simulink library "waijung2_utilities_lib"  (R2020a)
settings: Solver=VariableStepAuto  StartTime=0.0  StopTime=10.0  RelTol=1e-3
InitFcn:
  | waijung2_host_setup
undefined symbols (not defined in the file): BasicCustomCode, Button1, CircularBuffer, DataBuffer, fcn_call, float, int32_t, IRQ, IRQCustomCode, IRQCustomCode_ISR, OutputtoState, pointer_var, PointerBlock, Print, processing, Sensor1, Sensor2, Setup, statename, StringProcessing, Switch1, Switch2, Vector3x1, void

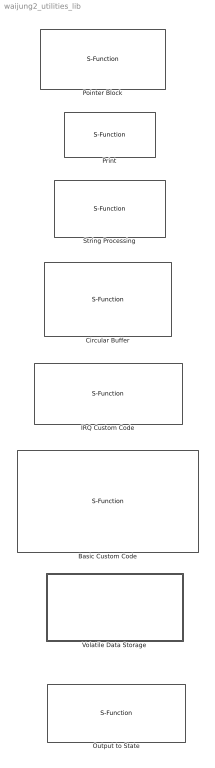
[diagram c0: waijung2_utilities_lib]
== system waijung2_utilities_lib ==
  Basic Custom Code : S-Function  FunctionName=waijung2_basic_customcode  Parameters=blockid,inputportcount,outputportcount,inputportdiminfo,outputportdiminfo,initialfuncallstr,enablefuncallstr,outputfuncallstr,disablefuncallstr,cinputportlabelstr,coutputportlabelstr,incfilestrarray,sampletime  SFunctionDeploymentMode=off  EnableBusSupport=off  mask(waijung2_basic_customcode){blockid=BasicCustomCode, maskdispname=BASIC CUSTOM CODE, inporttable={'Sensor1','double';'Sensor2','int8';'Switch1','single';'Switch2','uint16'}, outporttable={'Vector3x1','double','3x1';'Button1','int8','1x1';'5x20Matrix','int16','5x20'}, inputporttype=double,int8,single,uint16, cinputportlabel=Sensor1,Sensor2,Switch1,Switch2, cinputportlabelstr=["Sensor1","Sensor2","Switch1","Switch2"], inputportcount=4, inputporttypeid=[0  2  1  5], outputporttype=double:3x1,int8:1x1,int16:5x20, coutputportlabel=Vector3x1,Button1,5x20Matrix, coutputportlabelstr=["Vector3x1","Button1","5x20Matrix"], outputportcount=3, outputporttypeid=[0  2  4], filepath=, filenames=, incfilestrarray=, files=[], initialfuncallstr=, enablefuncallstr=, outputfuncallstr=, disablefuncallstr=, inputportdiminfo=[1  1  1  0;1  1  1  2;1  1  1  1;1  1  1  5], outputportdiminfo=[3  1  3  0;1  1  1  2;5   20  100    4], enablecustomportlabel=on, sampletime=-1}
      mask prompts: maskdispname "Mask display name"; inputporttype "Input port definition (data type) separted by comma e.g. double, single, double, uint8"; cinputportlabel "Custom input port labels (Ex. In1, In2, In3)"; outputporttype "Output port definition  (data type) separted by comma e.g. double, single, double, uint8"; coutputportlabel "Custom output port labels (Ex. Out1, Out2, Out3)"; initialfuncallstr "Initial function call string. Ex: init_funcname();"; enablefuncallstr "Enable function call string. Ex: enable_funcname();"; outputfuncallstr "Output function call string. Ex: output_funcname(in1,in2,in3,in4,out1,ou2,out3);"; disablefuncallstr "Disable function call string. Ex: disable_funcname();"; sampletime "Sample time (sec)"
      mask help: This block implements a basic custom code block. The Basic Custom Code Block supports 2-D input/output matrix/vector signals. The dimensions of input signals are automatically inherited from the supplied input signals. The dimensions of output signals must be implicitly defined using the following format. nRowsxnCols For examples: 4x5,int8,3x1 Define four-function prototypes: initial, enable, output, disable. o Initial function: An initial function will be called once at MCU start-up. o Enable function: An enable function will be called at system initialization and every time the block is enab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
      mask init:
      | waijung2_basic_customcode_callback('init');
  Circular Buffer : S-Function  FunctionName=waijung2_circular_buffer  Parameters=blockid,buffername,mode,inputporttype,inputportwidth,overwrite,datatypestring,portcount,packets,showindex,sampletime  SFunctionDeploymentMode=off  EnableBusSupport=off  mask(waijung2_circular_buffer){blockid=CircularBuffer, mode=Setup, buffernameedit=DataBuffer, buffernamepop=<empty>, buffername=DataBuffer, overwrite=on, showindex=off, packets=5, elements='%d, %f', inputporttype=[6 0], inputportwidth=[1 1], inputportlabel={'%d','%f'}, datatypestring=["int32_t","double"], portcount=2, sampletime=-1}
      mask prompts: buffernameedit "Buffer Name"; buffernamepop "Buffer Name"; overwrite "Allow overwrite buffer values"; showindex "Show read/wrting index"; packets "Length of the buffer"; elements "Input Format"; inputporttype "Input Port Type"; inputportwidth "Input Port Width"; inputportlabel "Input Port Label"; datatypestring "Data Type String"; portcount "Port Count"; sampletime "Sample time (sec)"
      mask help: Supported format: %u, %i, %o, %x: uint32 %d: int32 %e, %g, %f: single
      mask init:
      | waijung2_circular_buffer_callback('init');
  IRQ Custom Code : S-Function  FunctionName=waijung2_irq_customcode  Parameters=blockid,inputportcount,outputportcount,inputportdiminfo,outputportdiminfo,initialfuncallstr,enablefuncallstr,outputfuncallstr,disablefuncallstr,cinputportlabelstr,coutputportlabelstr,incfilestrarray,irqcntntbeforefcncall,irqcntntafterfcncall,editirqhandler,sampletime  SFunctionDeploymentMode=off  EnableBusSupport=off  mask(waijung2_irq_customcode){blockid=IRQCustomCode, maskdispname=IRQ CUSTOM CODE, inputporttype=, cinputportlabel=, cinputportlabelstr=[""], inputportcount=0, inputporttypeid=[-1], outputporttype=fcn_call, coutputportlabel=IRQ, coutputportlabelstr=["IRQ"], outputportcount=1, outputporttypeid=[9], filepath=, filenames=, incfilestrarray=, files=, initialfuncallstr=, enablefuncallstr=, outputfuncallstr=void IRQCustomCode_ISR(void), editirqhandler=off, irqhandlercontent=/* content before the code generated from the function-call subsystem */  %[function-call subsystem]  /* content after the function-callsubsystem */, irqcntntbeforefcncall=/* content before the code generated from the function-call subsystem */, irqcntntafterfcncall=/* content after the function-callsubsystem */, disablefuncallstr=, inputportdiminfo=[], outputportdiminfo=[1  1  1  9], enablecustomportlabel=on, sampletime=-1}
      mask prompts: maskdispname "Mask display name"; inputporttype "Input port definition (data type) separted by comma e.g. double, single, double, uint8"; cinputportlabel "Custom input port labels (Ex. In1, In2, In3)"; outputporttype "Output port definition  (data type) separted by comma e.g. double, single, double, uint8"; coutputportlabel "Custom output port labels (Ex. Out1, Out2, Out3)"; initialfuncallstr "Initial function call string. Ex: init_funcname();"; enablefuncallstr "Enable function call string. Ex: enable_funcname();"; outputfuncallstr "IRQ handler function prototype without semicolon. Ex: void IRQCustomCode_ISR(void)"; editirqhandler "Add additional content to the IRQ handler"; irqhandlercontent "IRQ handler content. Add the keyword '%[function-call subsystem]' to the place where the code generated from the function-call subsystem should be placed."; disablefuncallstr "Disable function call string. Ex: disable_funcname();"; sampletime "Sample time (sec)"
      mask help: This block implements a basic irq custom code block. Define four-function prototypes: initial, enable, disable. o Initial function: An initial function will be called once at MCU start-up. o Enable function: An enable function will be called at system initialization and every time the block is enabled. o Disable function: A disable function will be called at system termination and every time the block is disabled.
      mask init:
      | waijung2_irq_customcode_callback('init');
  Output to State : S-Function  FunctionName=waijung2_output_to_state  Parameters=blockid,sampletime,inputporttype,inputportwidth,statename  SFunctionDeploymentMode=off  EnableBusSupport=off  SFcnStateName=statename  mask(waijung2_output_to_state){blockid=OutputtoState, datawidth=1, datatype=double, statename=statename, enablestate=off, sampletime=-1, inputporttype=[0], inputportwidth=[1]}
      mask prompts: datawidth "Input data width"; datatype "Input data type"; statename "State name"; sampletime "Sample time"
      mask help: Output to State block is used to convert the simulink signal to Stateflow variable
      mask init:
      | waijung2_output_to_state_callback('init');
  Pointer Block : S-Function  FunctionName=waijung2_pointer  Parameters=blockid,vname,vtype,vsize,vinitialize,vvalue  SFunctionDeploymentMode=off  EnableBusSupport=off  mask(waijung2_pointer){vname=pointer_var, vtype=char, vsize=10, vinitialize=on, vvalue='aimagin', blockid=PointerBlock}
      mask prompts: vname "Pointer variable name"; vtype "Variable data type"; vsize "Variable size"; vinitialize "Initialize variable"; vvalue "Value"
      mask init:
      | waijung2_pointer_callback('init');
  Print : S-Function  FunctionName=waijung2_printf  Parameters=sampletime,sampletimestr,blockid,strinput,printfcn  SFunctionDeploymentMode=off  EnableBusSupport=off  mask(waijung2_printf){printfcn=<empty>, strinput=String Variable, sampletime=-1, blockid=Print, sampletimestr=2}
      mask prompts: printfcn "Print function"; strinput "String Input Type"; sampletime "Sample time (sec)"; blockid "Block ID"; sampletimestr "Sample time string"
      mask help: This block can be used to send formatted output to stdout
      mask init:
      | waijung2_printf_callback('init');
  String Processing : S-Function  FunctionName=waijung2_string_processing  Parameters=conf,stringfunction,stringformat,begindelimiter,enddelimiter,buffersize,enablestatus,datatypestring,inputporttype,inputportwidth,outputporttype,outputportwidth,optionstring,use_pointer,string_pointer,pointer_list,sampletime,blockid  SFunctionDeploymentMode=off  EnableBusSupport=off  mask(waijung2_string_processing){conf=processing, stringfunction=sprintf, stringformat='values = %d,%f', begindelimiter='', enddelimiter='', buffersize=64, enablestatus=off, use_pointer=off, pointer_list="", string_pointer=off, portpinstr=0, sampletime=-1, blockid=StringProcessing, inputporttype=[-1 -1], inputportwidth=[1 1], inputportlabel={'%d','%f'}, outputporttype=[3], outputportwidth=[64], outputportlabel={'Output'}, compat=0, optionstring=[], datatypestring=["int32_t","float"]}
      mask prompts: conf "Configuration"; stringfunction "Function"; stringformat "Format"; begindelimiter "Begin delimiter"; enddelimiter "End delimiter"; buffersize "Buffer size"; enablestatus "Enable output status"; use_pointer "Enable pointer"; pointer_list "Select pointer"; string_pointer "Output string pointer"; portpinstr "Port Pin String"; sampletime "Sample time (sec)"; blockid "Block ID"; inputporttype "Input Port Type"; inputportwidth "Input Port Width"; inputportlabel "Input Port Label"; outputporttype "Output Port Type"; outputportwidth "Output Port Width"; outputportlabel "Output port label"; compat "Compatibility (Reserved for future use)"; optionstring "String(s) to be passed to TLC"; datatypestring "Data types string"
      mask help: This block implements standard string formatting functions available in C Language. Supported format: %u, %i, %o, %x: uint32 %d: int32 %e, %g, %f: single %c: int8 %s: vector of data type uint8 Return: return number of success parameters.
      mask init:
      | waijung2_string_processing_callback('init');
  Volatile Data Storage : Subsystem

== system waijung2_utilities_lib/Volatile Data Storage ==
